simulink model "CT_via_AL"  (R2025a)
settings: Solver=VariableStepAuto  StartTime=0.0  StopTime=T  FixedStep=0.05  MaxStep=0.01  RelTol=1e-3  EnableMultiTasking=on
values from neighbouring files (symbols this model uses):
  k1 = 2*z*a    (= 9.8)    [CT_via_AL.m]
  k2 = (a^2-(om_d)^2)/v_d    (= 4.125)    [CT_via_AL.m]
  k3 = 2*z*a    (= 9.8)    [CT_via_AL.m]
  om_d = Omega    (= 4)    [CT_via_AL.m]
  Omega = 4    [CT_via_AL.m]
  R = [cos(theta), -sin(theta); sin(theta), cos(theta)]    [rotatePlanar.m]    (also in CT_via_AL.m = 2)
  theta_0 = theta_d0-eps    (= -1.42920367321)    [CT_via_AL.m]
  v_d = R*Omega    (= 8)    [CT_via_AL.m]
  x_0 = x_d0+eps    (= 5)    [CT_via_AL.m]
  y_0 = y_d0-eps    (= -3)    [CT_via_AL.m]
libraries: simulink x1

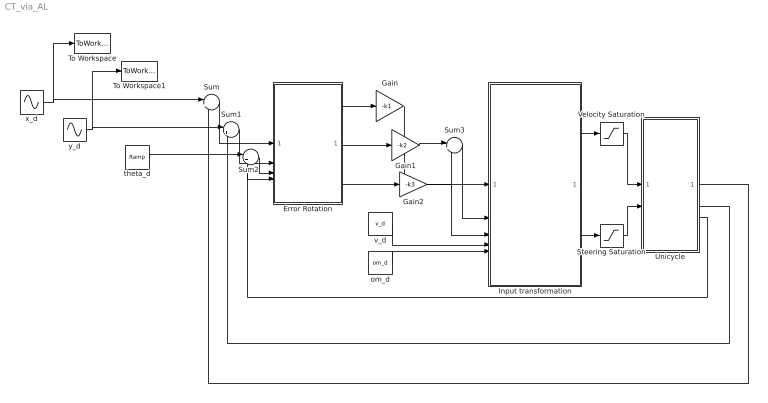
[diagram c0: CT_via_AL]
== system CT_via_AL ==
  Error Rotation : Subsystem
  Gain : Gain  Gain=-k1
  Gain1 : Gain  Gain=-k2
  Gain2 : Gain  Gain=-k3
  Input transformation : Subsystem
  Steering Saturation : Saturate  UpperLimit=1000  LowerLimit=-1000
  Sum : Sum  Inputs=|+-
  Sum1 : Sum  Inputs=|+-
  Sum2 : Sum  Inputs=|+-
  Sum3 : Sum  Inputs=|++
  To Workspace : ToWorkspace  VariableName=x_d  SampleTime=-1
  To Workspace1 : ToWorkspace  VariableName=y_d  SampleTime=-1
  Unicycle : Subsystem
  Velocity Saturation : Saturate  UpperLimit=1000  LowerLimit=-1000
  om_d : Constant  Value=om_d
  theta_d : simulink/Sources/Ramp  slope=Omega  start=0  InitialOutput=pi/2
  v_d : Constant  Value=v_d
  x_d : Sin  Amplitude=R  Frequency=Omega  Phase=pi/2  SampleTime=0
  y_d : Sin  Amplitude=R  Frequency=Omega  SampleTime=0
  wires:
  Sum/1 -> Error Rotation/1(x_d - x)
  Sum1/1 -> Error Rotation/2(y_d - y)
  Sum2/1 -> Error Rotation/3(theta_d - theta)
  Error Rotation/3(e3) -> Gain2/1
  Error Rotation/1(e1) -> Gain/1
  Gain/1 -> Input transformation/1(u1)
  Sum3/1 -> Input transformation/2(u2)
  x_d/1 -> Sum/1, To Workspace/1
  y_d/1 -> To Workspace1/1, Sum1/1
  theta_d/1 -> Sum2/1
  Input transformation/1(v) -> Velocity Saturation/1
  Input transformation/2(omega) -> Steering Saturation/1
  Unicycle/3(theta) -> Error Rotation/4(theta), Sum2/2
  Unicycle/2(y) -> Sum1/2
  Unicycle/1(x) -> Sum/2
  v_d/1 -> Input transformation/4(v_d)
  om_d/1 -> Input transformation/5(omega_d)
  Velocity Saturation/1 -> Unicycle/1(v)
  Steering Saturation/1 -> Unicycle/2(omega)
  Gain2/1 -> Input transformation/3(e3), Sum3/2
  Error Rotation/2(e2) -> Gain1/1
  Gain1/1 -> Sum3/1

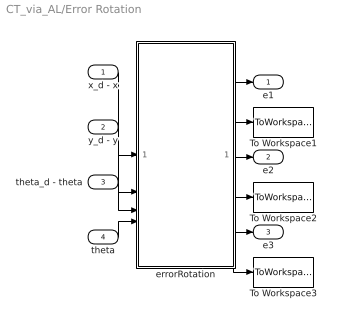
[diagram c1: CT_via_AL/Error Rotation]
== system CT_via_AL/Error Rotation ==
  x_d - x : Inport
  y_d - y : Inport  Port=2
  theta_d - theta : Inport  Port=3
  theta : Inport  Port=4
  To Workspace1 : ToWorkspace  VariableName=e1  SampleTime=-1
  To Workspace2 : ToWorkspace  VariableName=e2  SampleTime=-1
  To Workspace3 : ToWorkspace  VariableName=e3  SampleTime=-1
  errorRotation : MATLAB Function  TreatAsAtomicUnit=on
  e1 : Outport
  e2 : Outport  Port=2
  e3 : Outport  Port=3
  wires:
  x_d - x/1 -> errorRotation/1(u1)
  y_d - y/1 -> errorRotation/2(u2)
  theta_d - theta/1 -> errorRotation/3(u3)
  theta/1 -> errorRotation/4(theta)
  errorRotation/1(e1) -> To Workspace1/1, e1/1
  errorRotation/2(e2) -> To Workspace2/1, e2/1
  errorRotation/3(e3) -> To Workspace3/1, e3/1

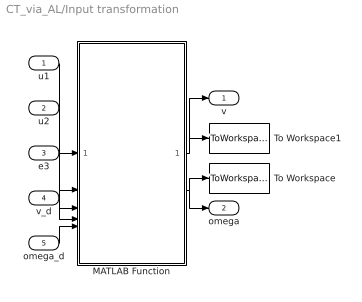
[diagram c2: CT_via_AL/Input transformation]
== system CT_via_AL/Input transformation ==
  u1 : Inport
  u2 : Inport  Port=2
  e3 : Inport  Port=3
  v_d : Inport  Port=4
  omega_d : Inport  Port=5
  MATLAB Function : MATLAB Function  TreatAsAtomicUnit=on
  To Workspace : ToWorkspace  VariableName=omega  SampleTime=-1
  To Workspace1 : ToWorkspace  VariableName=v  SampleTime=-1
  v : Outport
  omega : Outport  Port=2
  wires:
  u1/1 -> MATLAB Function/1(u1)
  u2/1 -> MATLAB Function/2(u2)
  v_d/1 -> MATLAB Function/4(v_d)
  e3/1 -> MATLAB Function/3(e3)
  omega_d/1 -> MATLAB Function/5(omega_d)
  MATLAB Function/1(v) -> To Workspace1/1, v/1
  MATLAB Function/2(omega) -> To Workspace/1, omega/1

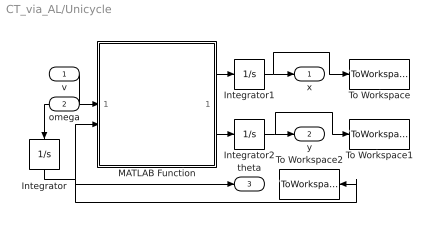
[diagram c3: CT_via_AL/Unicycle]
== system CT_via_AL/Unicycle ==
  v : Inport
  omega : Inport  Port=2
  Integrator : Integrator  InitialCondition=theta_0
  Integrator1 : Integrator  InitialCondition=x_0
  Integrator2 : Integrator  InitialCondition=y_0
  MATLAB Function : MATLAB Function  TreatAsAtomicUnit=on
  To Workspace : ToWorkspace  VariableName=x  SampleTime=-1
  To Workspace1 : ToWorkspace  VariableName=y  SampleTime=-1
  To Workspace2 : ToWorkspace  VariableName=theta  SampleTime=-1
  x : Outport
  y : Outport  Port=2
  theta : Outport  Port=3
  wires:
  omega/1 -> Integrator/1
  v/1 -> MATLAB Function/1(v)
  Integrator/1 -> MATLAB Function/2(theta), theta/1, To Workspace2/1
  MATLAB Function/1(xdot) -> Integrator1/1
  MATLAB Function/2(ydot) -> Integrator2/1
  Integrator1/1 -> x/1, To Workspace/1
  Integrator2/1 -> y/1, To Workspace1/1

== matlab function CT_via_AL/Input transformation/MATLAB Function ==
function [v,omega] = inputTransformation(u1, u2, e3, v_d, omega_d)

v = v_d.*cos(e3) - u1;
omega = omega_d - u2;

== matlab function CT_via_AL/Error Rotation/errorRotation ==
function [e1, e2, e3] = errorRotation(u1, u2, u3, theta)
%#codegen
mat = [cos(theta), sin(theta), 0;...
      -sin(theta), cos(theta), 0;...
                0,          0, 1];
e = mat*[u1; u2; u3];

e1 = e(1);
e2 = e(2);
e3 = e(3);

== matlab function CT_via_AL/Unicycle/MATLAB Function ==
function [xdot, ydot] = unicicle(v, theta)

xdot = v.*cos(theta);
ydot = v.*sin(theta);
